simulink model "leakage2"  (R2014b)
settings: Solver=ode45  StartTime=0.0  StopTime=10.0  RelTol=1e-3
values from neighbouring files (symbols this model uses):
  ampl = 1    [abtast_rate_1.m]    (also in ad_test_12.m; ad_test_2.m; ad_test_3.m; fft_1.m = 10)
  fsig = 100    [abtast_rate_1.m]    (also in ad_test_12.m = ',num2str(fsig),'; ad_test_2.m = ',num2str(fsig),'; ad_test_3.m = ',num2str(fsig),'; leakage_2.m = 100.5)
  N = 4*1024    (= 4096)    [ad_test_12.m]    (also in ad_test_2.m; ad_test_3.m; DA_wandler_spektr_1.m = 1000; DA_wandler_spektr_2.m = 1024)
  phi = pi/3    (= 1.0471975512)    [fft_1.m]    (also in fft_2.m; fourier_transf_puls_3.m = phi(:,:,end); fourier_transf_puls_4.m = phi(:,:,end); leakage_1.m)
  pw = sum(hanning(N).^2)/N    [leakage_2.m]    (also in leakage_3.m; leakage_4.m; welch_1.m = sum(hamming(nfft).^2)/nfft; zero_padd2.m = sum(hamming(N).^2)/N)
  Ts = 1/fs    (= 0.00025)    [abtast_rate_1.m]    (also in ad_test_12.m = 0.0009765625; ad_test_2.m = 0.00048828125; ad_test_3.m = 0.00048828125; DA_wandler_spektr_1.m = 0.01)
undefined symbols (not defined in the file or in its folder): get
libraries: dspspect3 x2, dspsigops x2, dspsnks4 x1

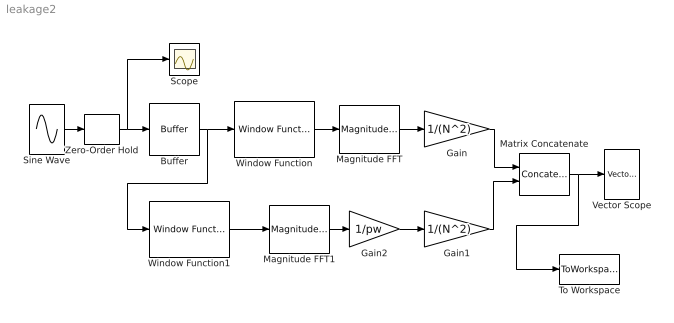
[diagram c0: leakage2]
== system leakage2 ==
  Buffer : Buffer  N=N  TreatMby1Signals=One channel
  Gain : Gain  Gain=1/(N^2)
  Gain1 : Gain  Gain=1/(N^2)
  Gain2 : Gain  Gain=1/pw
  Magnitude FFT : dspspect3/Magnitude FFT  mag_or_magsq=Magnitude squared  FFTImplementation=Auto  fftLenInherit=on  fftsize=256  WrapInput=on
  Magnitude FFT1 : dspspect3/Magnitude FFT  mag_or_magsq=Magnitude squared  FFTImplementation=Auto  fftLenInherit=on  fftsize=256  WrapInput=on
  Matrix Concatenate : Concatenate  Mode=Multidimensional array  ConcatenateDimension=2
  Scope : Scope
  Sine Wave : Sin  Amplitude=ampl  Frequency=2*pi*fsig  Phase=phi  SampleTime=0
  To Workspace : ToWorkspace  VariableName=Y  SampleTime=-1
  Vector Scope : dspsnks4/Vector Scope  ScopeProperties=on  Domain=Frequency  HorizSpan=1  DisplayProperties=off  AxisGrid=on  Memory=off  FrameNumber=on  AxisLegend=off  AxisZoom=off  OpenScopeAtSimStart=on  OpenScopeImmediately=off  FigPos=get(0,'defaultfigureposition')  AxisProperties=off  XUnits=Hertz  XRange=[0...Fs]  InheritXIncr=on  XIncr=1  XLabel=Time  XLimit=Auto  XMin=0  XMax=1  XStart=0  YUnits=dB  YLabel=Leistung in dB  LineProperties=off  XAxisParamsVer=6.9
  Window Function : dspsigops/Window Function  winmode=Apply window to input  wintype=Boxcar  sampmode=Continuous  samptime=1  N=64  Rs=50  beta=10  winsamp=Symmetric  UserWindow=fenster  OptParams=on  UserParams={'symmetric'}  RowConvenienceOn=on  dataType=double  isSigned=on  wordLen=16  udDataType=sfix(16)  fracBitsMode=Best precision  numFracBits=15  roundingMode=Floor  overflowMode=off  numSidelobes=4  sidelobeLevel=-30
  Window Function1 : dspsigops/Window Function  winmode=Apply window to input  wintype=Hanning  sampmode=Continuous  samptime=1  N=64  Rs=50  beta=10  winsamp=Symmetric  UserWindow=fenster  OptParams=on  UserParams={'symmetric'}  RowConvenienceOn=on  dataType=double  isSigned=on  wordLen=16  udDataType=sfix(16)  fracBitsMode=Best precision  numFracBits=15  roundingMode=Floor  overflowMode=off  numSidelobes=4  sidelobeLevel=-30
  Zero-Order Hold : ZeroOrderHold  SampleTime=Ts
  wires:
  Sine Wave/1 -> Zero-Order Hold/1
  Zero-Order Hold/1 -> Scope/1, Buffer/1
  Buffer/1 -> Window Function1/1, Window Function/1
  Magnitude FFT/1 -> Gain/1
  Window Function/1 -> Magnitude FFT/1
  Magnitude FFT1/1 -> Gain2/1
  Gain1/1 -> Matrix Concatenate/2
  Window Function1/1 -> Magnitude FFT1/1
  Gain/1 -> Matrix Concatenate/1
  Matrix Concatenate/1 -> To Workspace/1, Vector Scope/1
  Gain2/1 -> Gain1/1
